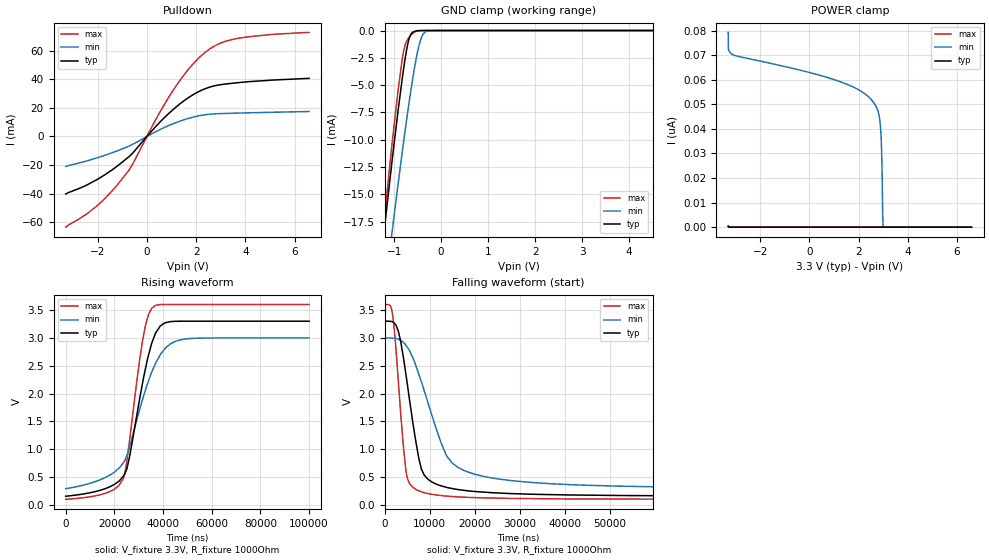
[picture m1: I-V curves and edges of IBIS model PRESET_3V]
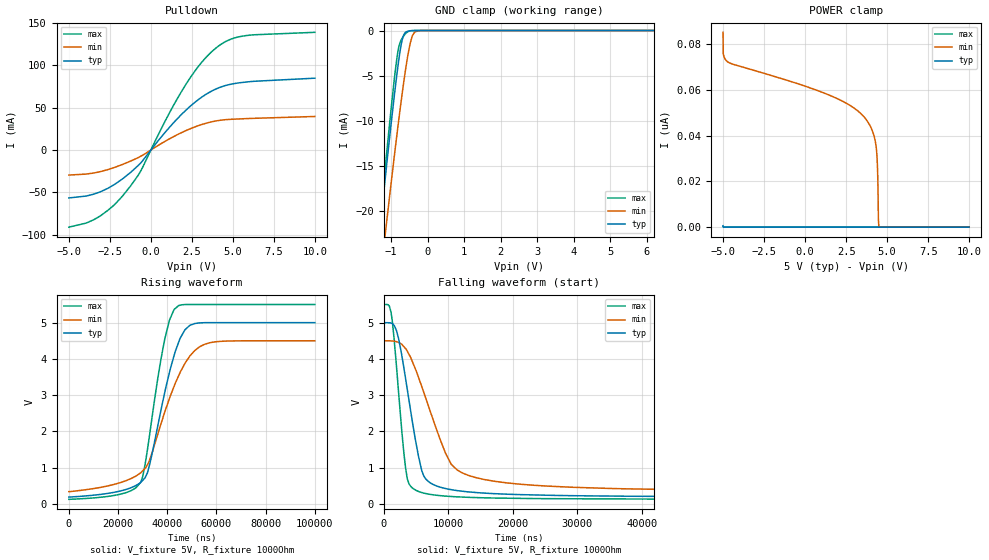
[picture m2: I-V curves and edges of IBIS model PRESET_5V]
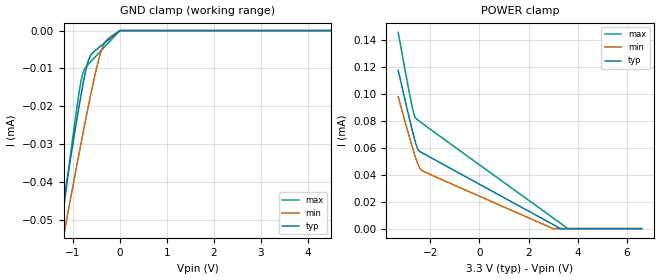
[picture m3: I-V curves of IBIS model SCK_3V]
| Texas Instruments Incorporated
| Low-Noise Clock Jitter Cleaner with Dual Loop PLLs
| Marketing part#   Voltage Range   Package-type   #pins/pkg drawing
| TPS65310   3.0V - 3.6V   LLP   64-pin SQ
[IBIS Ver]   4.1
[File name]   tps65310.ibs
[File Rev]   1.0
[Date]   05/14/2013
[Source]   Model built from spectre simulations at:
   Texas Instruments Incorporated.
   Analog-eLab, HPA
   12500 TI Blvd
   Dallas, TX -75243
   For Support e-mail: elab_ibis@list.ti.com
[Notes]   Revision History
   Rev 1.0: 05/14/2013
   -Update OSCIN and CLKIN input buffer models
   -Combined Pullup/Pulldown non-monotonic for SDO_5V, SDO_3V models
   - ccomp values are based on PVT settings:
   MIN: Low Voltage, High Temperature, Weak Process
   TYP: Nominal Voltage, Nominal Temperature, Nominal Process
   MAX: High Voltage, Low Temperature, Fast Process
   - C_comp although listed in numerical order of value are obtained from varying PVT conditions.
   For PVT conditions for each specific value, refer to the buffer description under respective [Model].
   IBIS model user is responsible for using appropriate C_comp to simulate for Signal Integrity.
[Disclaimer]  This model is designed as an aid for customers of Texas Instruments
 TI and its licensors and suppliers make no warranties, either expressed
 or implied, with respect to this  model, including the warranties of
 merchantability or fitness for a particular purpose.
 The model is provided solely on an "as is" basis. The entire risk as to
 its quality and performance is with the customer.
[Copyright] (C)Copyright 2013 Texas Instruments Incorporated.
   All rights reserved.
[Component]   TPS65310RVJ
[Manufacturer]  Texas Instruments Incorporated
[Package]   |56-pin QFN package
|   typ   min   max
R_pkg   0.005   0.005   0.005
L_pkg   0.2nH   0.2nH   0.2nH
C_pkg   0.6pF   0.6pF   0.6pF
[Pin]   signal_name   model_name   R_pin   L_pin   C_pin
1   VSSENSE   NC
2   VIN   NC
3   GPFET   NC
4   VINPROT   NC
5   HSCTRL   NC
6   HSSENSE   NC
7   WAKE   NC
8   EXTSUP   NC
9   VREG   NC
10   BOOT1   NC
11   GU   NC
12   PH1   NC
13   GL   NC
14   PGND1   NC
15   S1   NC
16   S2   NC
17   VMON1   NC
18   COMP1   NC
19   VSENSE1   NC
20   COMP5   NC
21   VSENSE5   NC
22   PGND5   NC
23   PH5   NC
24   VBOOST   NC
25   VT_REF   NC
26   PRESN   NC
27   RESN   NC
28   IRQ   NC
29   BOOT2   NC
30   VSUP2   NC
31   PH2   NC
32   PGND2   NC
33   VMON2   NC
34   COMP2   NC
35   VSENSE2   NC
36   VSENSE3   NC
37   COMP3   NC
38   VMON3   NC
39   PGND3   NC
40   PH3   NC
41   VSUP3   NC
42   BOOT3   NC
43   WD   WD
44   CSN   CSN
45   SDI   SCK
46   SCK   SCK
47   SDO   SDO
48   VIO   NC
49   HSPWM   SCK
50   VSUP4   NC
51   LDO   NC
52   VSENSE4   NC
53   VREF   NC
54   VT   NC
55   DVDD   POWER
56   GND   GND
[Model Selector] PRESET
PRESET_3V   PRESET 3.3V Open Drain Output
PRESET_5V   PRESET 5V Open Drain Output
[Model Selector] RESET
RESET_3V   RESET 3.3V Open Drain Output
RESET_5V   RESET 5V Open Drain Output
[Model Selector] SCK
SCK_3V   SDI 3.3V Input
SCK_5V   SDI 5V Input
[Model Selector] CSN
CSN_3V   SDI 3.3V Input
CSN_5V   SDI 5V Input
[Model Selector] WD
WD_3V   WD 3.3V Input
WD_5V   WD 5V Input
[Model Selector] SDO
SDO_3V   SDO 3.3V Output
SDO_5V   SDO 5V Output
| Models and submodels in the file (12): PRESET_3V (Open_drain), PRESET_5V (Open_drain), RESET_3V (Open_drain), RESET_5V (Open_drain), SCK_3V (Input), SCK_5V (Input), WD_3V (Input), WD_5V (Input), CSN_3V (Input), CSN_5V (Input), SDO_3V (Output), SDO_5V (Output)
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|   Buffer Models
[Model]   PRESET_3V
Model_type   Open_drain
Polarity   Non-Inverting
Vmeas = 1.65
Vref = 3.3
Cref = 15pF
Rref = 1000
|   typ   min   max
|   (slow PVT)   (Fast PVT)   (nom PVT)
C_comp   0.457p   0.385p   0.489p
|C_comp (hi state)   1.424p   1.168p   1.512p
|C_comp (low state)   0.457p   0.385p   0.489p
[Voltage Range]   3.3   3   3.6
[Temperature Range]   27   175   -40
[Pullup Reference]   3.3   3   3.6
[Pulldown Reference]   -0   -0   -0
[Power Clamp Reference]   3.3   3   3.6
[GND Clamp Reference]   -0   -0   -0
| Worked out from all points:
|   slope of the pulldown table from 0 to 0.495 V, typ, clamps not added: 52.8 ohm
|   GND clamp passes 1 mA (typ) near -0.70 V on its own axis
|   falling waveform, V_fixture 3.3V, R_fixture 1000Ohm: 20-80 % time 3.62us typ, 7.05us min, 2.07us max; typ from 3.3 V to 0.159 V
|   rising waveform, V_fixture 3.3V, R_fixture 1000Ohm: 20-80 % time 8.09us typ, 11.4us min, 6.26us max; typ from 0.158 V to 3.3 V
[Pulldown]
|   Voltage   I(typ)   I(min)   I(max)
-3.3V     -40.22mA   -20.93mA   -63.36mA
-2.023V   -30.08mA   -14.94mA   -48.4mA
-1.429V   -23.54mA   -11.5mA    -38.31mA
-815.1mV  -15.36mA   -7.411mA   -25.51mA
-547.8mV  -11.06mA   -5.234mA   -18.35mA
531.3mV   10.03mA    4.774mA    17.04mA
1.076V    18.95mA    8.94mA     32.44mA
1.739V    27.67mA    12.86mA    47.92mA
2.363V    33.29mA    15.14mA    58.64mA
2.917V    35.92mA    15.9mA     64.61mA
3.61V     37.38mA    16.26mA    68.21mA
6.59V     40.56mA    17.41mA    72.71mA
[GND Clamp]
|   Voltage   I(typ)   I(min)   I(max)
-3.3V     -112.4mA   -105.1mA   -127.4mA
-1.27V    -20.52mA   -26.45mA   -19.78mA
-1.033V   -11.5mA    -18.04mA   -9.879mA
-914.1mV  -7.251mA   -13.97mA   -5.371mA
-795.3mV  -3.393mA   -10.07mA   -1.813mA
-686.4mV  -818.2uA   -6.702mA   -646uA
-587.4mV  -112uA     -3.938mA   -194.6uA
-508.2mV  -24.91uA   -2.071mA   -41.17uA
-429mV    -4.844uA   -750.9uA   -4.95uA
-379.5mV  -1.547uA   -305.8uA   -1.011uA
-270.6mV  -103.2nA   -26.66uA   -23.76nA
6.59V     0A         0A         0A
[POWER Clamp]
|   Voltage   I(typ)   I(min)   I(max)
-3.3V     487.5pA    79.27nA    133.5pA
-3.29V    243.8pA    72.38nA    66.75pA
-3.112V   0A         70.15nA    0A
1.096V    0A         59.73nA    0A
2.591V    0A         50.98nA    0A
2.779V    0A         47.44nA    0A
2.888V    0A         41.01nA    0A
2.937V    0A         30.04nA    0A
2.957V    0A         20.57nA    0A
2.977V    0A         5.48nA     0A
2.996V    0A         0A         0A
6.59V     0A         0A         0A
[Ramp]
R_load = 1000
|   typ   min   max
dV/dt_r   1.88533/8.08802e-06   1.62387/1.14437e-05   2.0991/6.25912e-06
dV/dt_f   1.88442/3.617e-06   1.61946/7.05222e-06   2.09893/2.06537e-06
[Falling Waveform]
V_fixture = 3.3V
V_fixture_min = 3V
V_fixture_max = 3.6V
R_fixture = 1000Ohm
C_fixture = 0F
|   Time   V(typ)   V(min)   V(max)
0s        3.3V       3V         3.6V
1.774us   3.288V     2.995V     3.401V
3.025us   3.116V     2.976V     2.206V
4.746us   2.316V     2.862V     588mV
7.683us   794.4mV    2.317V     249.9mV
9.329us   482.8mV    1.905V     210.4mV
13.71us   316.9mV    885.4mV    160mV
20.16us   241.6mV    548.8mV    132.4mV
43.06us   178.4mV    359.5mV    108.4mV
100us     159.3mV    300.8mV    101.8mV
[Rising Waveform]
V_fixture = 3.3V
V_fixture_min = 3V
V_fixture_max = 3.6V
R_fixture = 1000Ohm
C_fixture = 0F
|   Time   V(typ)   V(min)   V(max)
0s        157.8mV    293.5mV    101.5mV
17.77us   319.4mV    527.4mV    233.6mV
23.77us   521.8mV    764.2mV    483.4mV
26.31us   884.4mV    1.052V     1.185V
31.59us   2.19V      1.897V     2.952V
33.99us   2.685V     2.225V     3.417V
35.44us   2.916V     2.396V     3.538V
38.93us   3.218V     2.703V     3.598V
47.06us   3.3V       2.965V     3.6V
100us     3.3V       3V         3.6V
[Model]   PRESET_5V
Model_type   Open_drain
Polarity   Non-Inverting
Vmeas = 2.5
Vref = 2.5
Cref = 15pF
Rref = 1000
|   typ   min   max
|   (slow PVT)   (Fast PVT)   (nom PVT)
C_comp   0.405p   0.348p   0.442p
|C_comp (hi state)   1.201p   1.032p   1.317p
|C_comp (low state)   0.405p   0.348p   0.442p
[Voltage Range]   5   4.5   5.5
[Temperature Range]   27   175   -40
[Pullup Reference]   5   4.5   5.5
[Pulldown Reference]   -0   -0   -0
[Power Clamp Reference]   5   4.5   5.5
[GND Clamp Reference]   -0   -0   -0
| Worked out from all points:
|   slope of the pulldown table from 0 to 0.75 V, typ, clamps not added: 41.4 ohm
|   GND clamp passes 1 mA (typ) near -0.69 V on its own axis
|   falling waveform, V_fixture 5V, R_fixture 1000Ohm: 20-80 % time 2.74us typ, 5.2us min, 1.58us max; typ from 5 V to 0.19 V
|   rising waveform, V_fixture 5V, R_fixture 1000Ohm: 20-80 % time 9.48us typ, 12.9us min, 7.39us max; typ from 0.189 V to 5 V
[Pulldown]
|   Voltage   I(typ)   I(min)   I(max)
-5V       -56.66mA   -29.63mA   -91.15mA
-3.965V   -54.45mA   -28.49mA   -86.44mA
-3.17V    -50.06mA   -25.98mA   -78.92mA
-1.715V   -33.93mA   -16.99mA   -54.11mA
-620mV    -15.39mA   -7.425mA   -24.82mA
850mV     20.44mA    10.07mA    33.46mA
2.11V     46.58mA    22.68mA    76.81mA
3.07V     62.01mA    29.89mA    102.9mA
4V        72.33mA    34.41mA    121mA
4.84V     77.52mA    36.17mA    130.6mA
5.68V     79.99mA    36.92mA    134.8mA
9.985V    84.78mA    39.55mA    138.9mA
[GND Clamp]
|   Voltage   I(typ)   I(min)   I(max)
-5V       -209.6mA   -185mA     -240mA
-1.64V    -35.7mA    -40.23mA   -36.73mA
-1.25V    -19.96mA   -25.89mA   -19.18mA
-1.115V   -14.77mA   -21.07mA   -13.47mA
-905mV    -7.12mA    -13.8mA    -5.271mA
-800mV    -3.691mA   -10.33mA   -2.112mA
-725mV    -1.674mA   -7.953mA   -1.086mA
-665mV    -639.7uA   -6.147mA   -679.4uA
-545mV    -84.71uA   -2.923mA   -153.9uA
-410mV    -6.722uA   -555.5uA   -6.46uA
-200mV    -16.47nA   -5.701uA   0A
9.985V    0A         0A         0A
[POWER Clamp]
|   Voltage   I(typ)   I(min)   I(max)
-5V       628.4pA    85.13nA    199.5pA
-4.985V   314.2pA    75.63nA    99.76pA
-4.7V     0A         72.13nA    0A
1.435V    0A         57.8nA     0A
3.67V     0A         47.49nA    0A
4.12V     0A         41.65nA    0A
4.33V     0A         34.98nA    0A
4.405V    0A         27.05nA    0A
4.435V    0A         19.08nA    0A
4.465V    0A         3.271nA    0A
4.495V    0A         0A         0A
9.985V    0A         0A         0A
[Ramp]
R_load = 1000
|   typ   min   max
dV/dt_r   2.88656/9.47786e-06   2.49662/1.29369e-05   3.22399/7.38858e-06
dV/dt_f   2.88575/2.74355e-06   2.49263/5.19602e-06   3.22384/1.58452e-06
[Falling Waveform]
V_fixture = 5V
V_fixture_min = 4.5V
V_fixture_max = 5.5V
R_fixture = 1000Ohm
C_fixture = 0F
|   Time   V(typ)   V(min)   V(max)
0s        5V         4.5V       5.5V
880.3ns   4.996V     4.499V     5.458V
1.345us   4.973V     4.494V     5.042V
2.309us   4.569V     4.456V     3.105V
3.149us   3.744V     4.336V     1.389V
3.664us   3.164V     4.212V     697.4mV
6.159us   802.1mV    3.112V     301.2mV
10.5us    393.4mV    1.089V     205.1mV
17.27us   282.7mV    622.5mV    162.6mV
100us     190.4mV    345.5mV    126.9mV
[Rising Waveform]
V_fixture = 5V
V_fixture_min = 4.5V
V_fixture_max = 5.5V
R_fixture = 1000Ohm
C_fixture = 0F
|   Time   V(typ)   V(min)   V(max)
0s        189.1mV    338.9mV    126.7mV
21.22us   361.2mV    593.6mV    272.4mV
29.22us   594.2mV    857.8mV    594.9mV
31.99us   861.9mV    1.087V     1.51V
39.01us   3.078V     2.536V     4.549V
40.9us    3.623V     2.906V     5.066V
44.67us   4.464V     3.539V     5.471V
49.2us    4.926V     4.079V     5.5V
57.27us   4.999V     4.445V     5.5V
100us     5V         4.5V       5.5V
[Model]   SCK_3V
Model_type   Input
Vinl = .8
Vinh = 2.
|   typ   min   max
C_comp   0.01p   0.01p   0.01p
[Voltage Range]   3.3   3   3.6
[Temperature Range]   27   175   -40
[Power Clamp Reference]   3.3   3   3.6
[GND Clamp Reference]   -0   -0   -0
[GND Clamp]
|   Voltage   I(typ)   I(min)   I(max)
-3.3V     -216uA     -198.3uA   -263.1uA
-1.36V    -58.01uA   -65.01uA   -63.4uA
-1.28V    -51.7uA    -59.68uA   -55.44uA
-1.181V   -43.87uA   -53.04uA   -45.57uA
-894.3mV  -21.84uA   -34.08uA   -18.43uA
-785.4mV  -14.19uA   -27.07uA   -11.15uA
-686.4mV  -8.557uA   -20.86uA   -9.07uA
-627mV    -6.642uA   -17.25uA   -8.273uA
-389.4mV  -3.897uA   -5.064uA   -5.137uA
-270.6mV  -2.707uA   -2.371uA   -3.569uA
-3.3mV    -32.02nA   -25.49nA   -42.57nA
6.59V     0A         0A         0A
[POWER Clamp]
|   Voltage   I(typ)   I(min)   I(max)
-3.3V     117.8uA    98.08uA    145.9uA
-2.934V   88.75uA    73.86uA    109.3uA
-2.716V   72.23uA    60.09uA    89.22uA
-2.617V   65.32uA    54.23uA    82.99uA
-2.528V   60.21uA    49.44uA    81.16uA
-2.458V   57.98uA    46.34uA    80.17uA
-2.34V    56.49uA    43.28uA    78.53uA
-825mV    41.29uA    30.78uA    58.39uA
2.996V    3.038uA    27.9nA     7.963uA
3.293V    65.05nA    0A         4.045uA
3.59V     0A         0A         125.7nA
6.59V     0A         0A         0A
